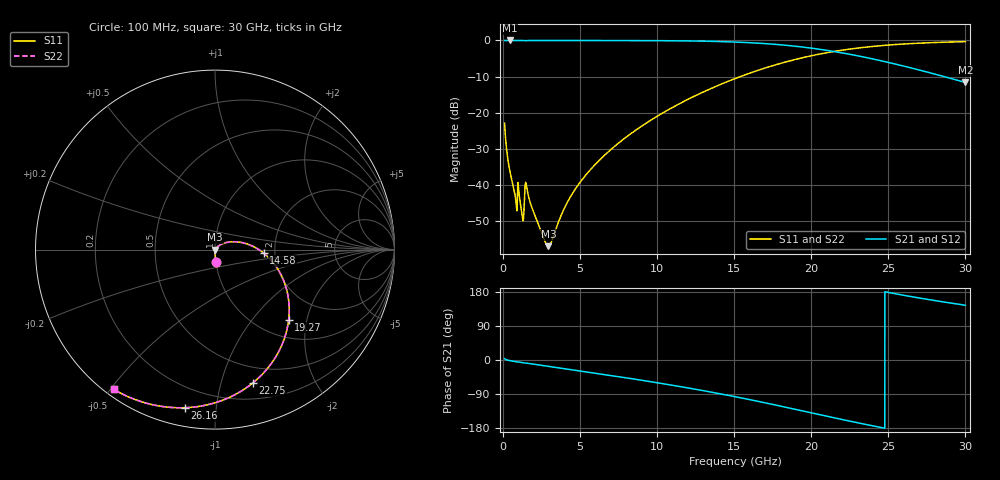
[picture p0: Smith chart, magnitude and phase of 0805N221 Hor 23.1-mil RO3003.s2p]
# GHz S MA R 50
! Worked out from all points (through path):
!   3201 points, 100 MHz to 30 GHz, reference 50 ohm
!   highest |S21| = -0.01 dB at 436.4 MHz (marker M1); lowest = -11.6 dB at 30 GHz (marker M2)
!   group delay of S21, straight-line fit = 20.9 ps
!   lowest |S11| = -56.9 dB at 2.941 GHz (marker M3), VSWR 1.00, Z = 50.1 - j0.0451 ohm
!   |S11| at or under -10 dB: start of sweep to 15.4 GHz
!   |S22| runs from -56.9 to -0.3 dB; largest |S21 - S12| = 0
!   S11 on the Smith chart (normalised r, x): 100 MHz: 1.00, -0.14; 14.58 GHz: 1.74, -0.07; 19.27 GHz: 1.36, -1.56; 22.75 GHz: 0.35, -1.27; 26.16 GHz: 0.09, -0.82; 30 GHz: 0.02, -0.51
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0.1  0.07166 -86.3  0.9972 3.5  0.9972 3.5  0.07166 -86.3
0.436375  0.01582 -89.8  0.9994 -1.6  0.9994 -1.6  0.01582 -89.8
0.77275  0.007364 -87.8  0.9992 -4.0  0.9992 -4.0  0.007364 -87.8
1.07175  0.006622 -83.5  0.9985 -5.8  0.9985 -5.8  0.006622 -83.5
1.211906  0.004158 -75.4  0.9984 -6.7  0.9984 -6.7  0.004158 -75.4
1.557625  0.008778 -72.1  0.996 -8.4  0.996 -8.4  0.008778 -72.1
1.856625  0.004957 -81.9  0.9983 -10.3  0.9983 -10.3  0.004957 -81.9
2.613469  0.001881 -57.6  0.9985 -14.8  0.9985 -14.8  0.001881 -57.6
2.9405  0.001423 -18.4  0.9985 -16.7  0.9985 -16.7  0.001423 -18.4
4.089781  0.005329 48.8  0.9982 -23.5  0.9982 -23.5  0.005329 48.8
5.089563  0.01156 51.6  0.9979 -29.4  0.9979 -29.4  0.01156 51.6
7.20125  0.03373 44.1  0.9969 -42.1  0.9969 -42.1  0.03373 44.1
10.06978  0.09116 27.7  0.9926 -60.5  0.9926 -60.5  0.09116 27.7
14.58281  0.2709 -4.0  0.9578 -93.1  0.9578 -93.1  0.2709 -4.0
15.05  0.2965 -7.6  0.95 -96.8  0.95 -96.8  0.2965 -7.6
17.05891  0.4189 -24.2  0.9022 -113.5  0.9022 -113.5  0.4189 -24.2
19.27338  0.5661 -43.5  0.8176 -132.9  0.8176 -132.9  0.5661 -43.5
20.03956  0.6162 -50.3  0.7806 -139.8  0.7806 -139.8  0.6162 -50.3
22.74925  0.7715 -74.0  0.6284 -163.5  0.6284 -163.5  0.7715 -74.0
25.01978  0.8638 -92.4  0.4953 178.1  0.4953 178.1  0.8638 -92.4
26.15972  0.8971 -100.9  0.433 169.6  0.433 169.6  0.8971 -100.9
30  0.9621 -125.9  0.262 144.5  0.262 144.5  0.9621 -125.9
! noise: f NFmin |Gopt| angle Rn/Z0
0.1  0.0003684  0.8385  0.6356  0.0004829
3.417  0.00546  0.6657  19.4  0.003047
6.743  0.009128  0.624  37.57  0.004093
10.06  0.01285  0.616  54.55  0.004993
13.39  0.01703  0.6258  70.26  0.005846
16.7  0.02203  0.6481  84.7  0.006734
20.03  0.02844  0.6807  98.2  0.007744
23.35  0.03711  0.722  111  0.008949
26.67  0.04963  0.7703  123.7  0.01039
30  0.06886  0.8221  136.3  0.0119
